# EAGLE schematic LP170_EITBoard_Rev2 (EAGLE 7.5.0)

## Sheet 1 of 9: Arduino Mega 2560 Board Connections
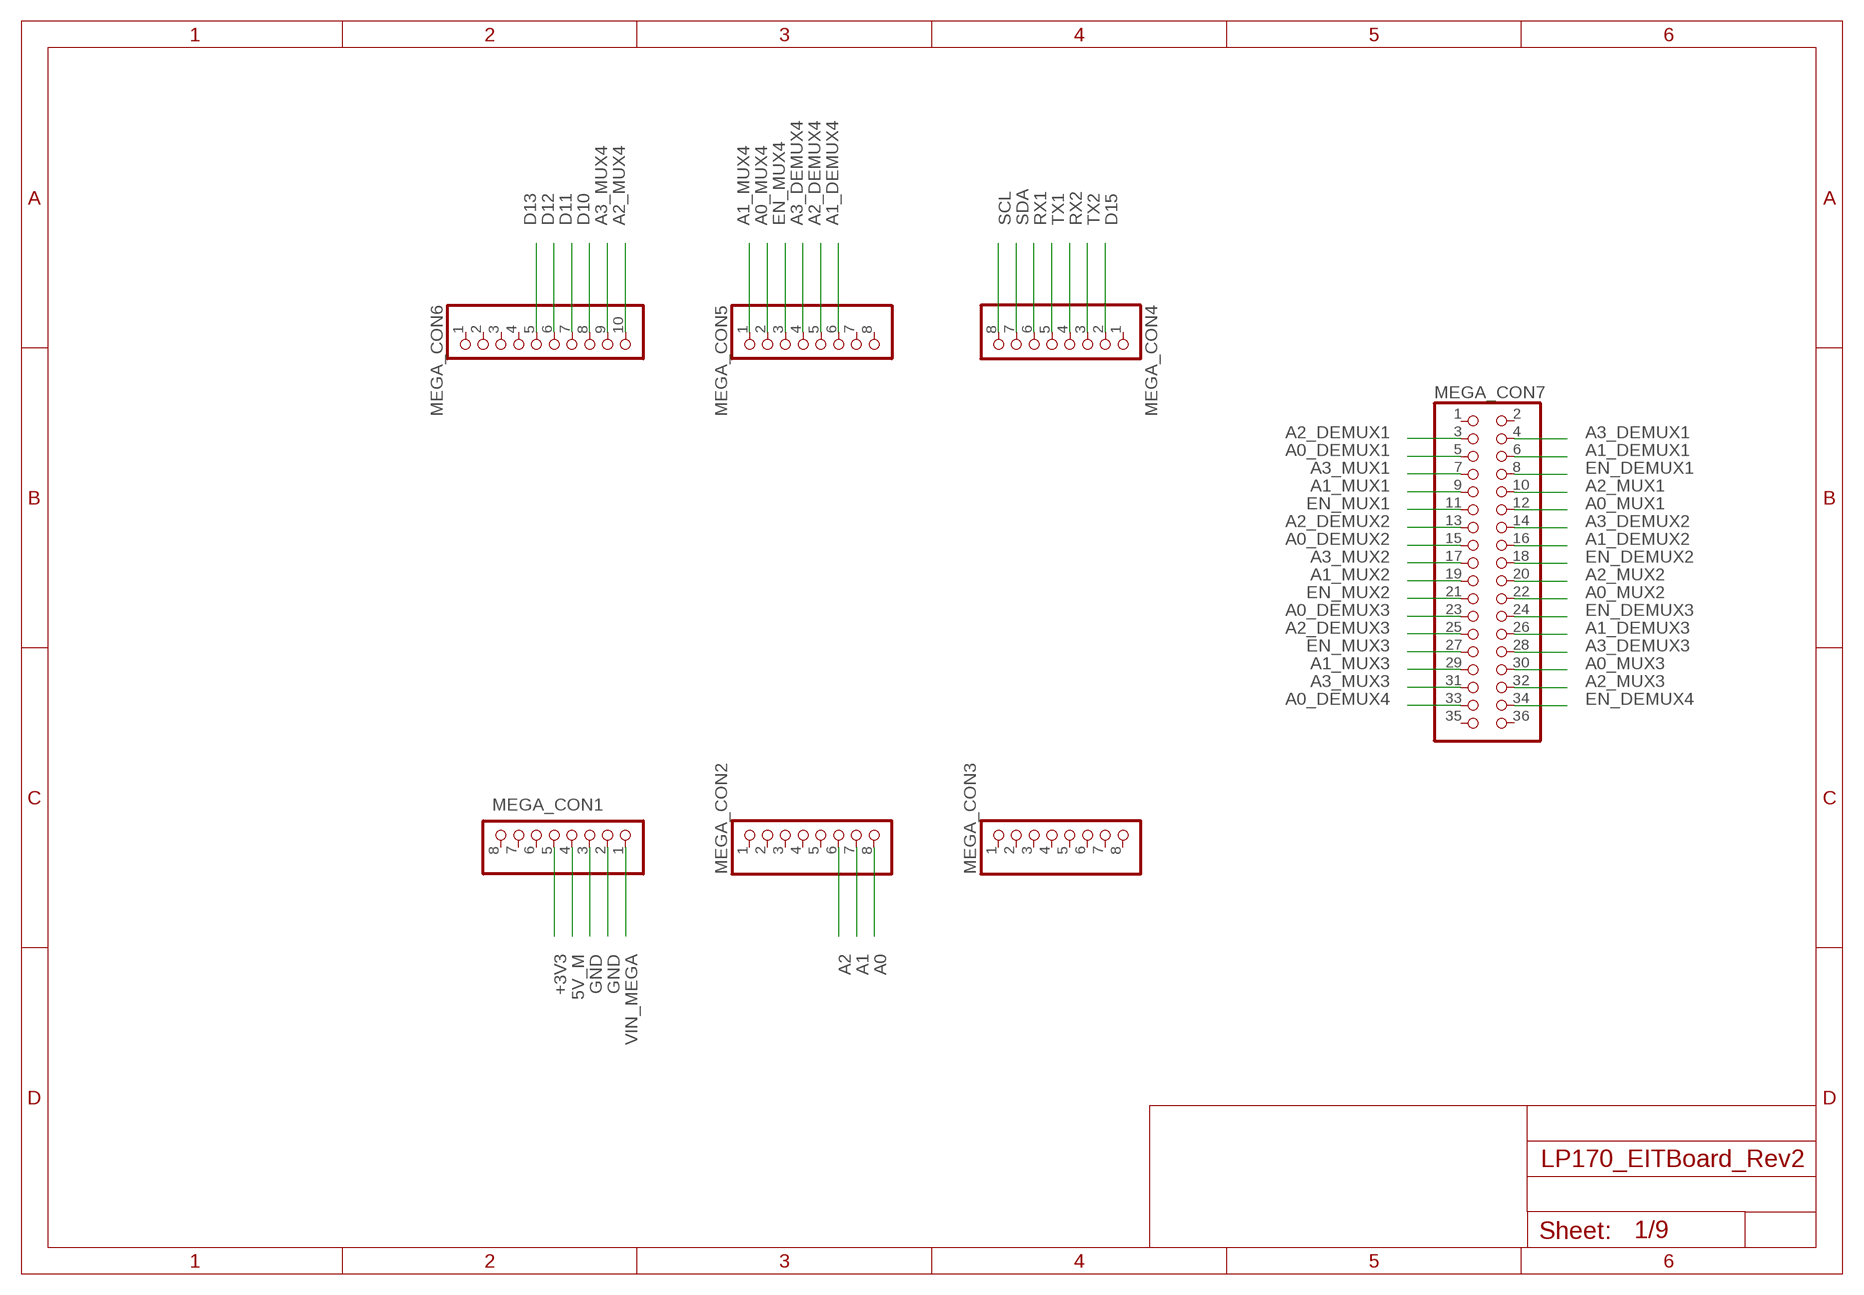
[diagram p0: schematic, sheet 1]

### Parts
MEGA_CON1  PINHD-1X8BIG  [1X08-BIG]
MEGA_CON2  PINHD-1X8BIG  [1X08-BIG]
MEGA_CON3  PINHD-1X8BIG  [1X08-BIG]
MEGA_CON4  PINHD-1X8BIG  [1X08-BIG]
MEGA_CON5  PINHD-1X8BIG  [1X08-BIG]
MEGA_CON6  PINHD-1X10  [1X10-BIG]
MEGA_CON7  PINHD-2X18  [2X18]

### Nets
5V_M: MEGA_CON1.4
+3V3: MEGA_CON1.5 ; also sheet 3,9
A0: MEGA_CON2.8
A0_DEMUX1: MEGA_CON7.5 ; also sheet 4
A0_DEMUX2: MEGA_CON7.15 ; also sheet 4
A0_DEMUX3: MEGA_CON7.23 ; also sheet 4
A0_DEMUX4: MEGA_CON7.33 ; also sheet 4
A0_MUX1: MEGA_CON7.12 ; also sheet 5
A0_MUX2: MEGA_CON7.22 ; also sheet 5
A0_MUX3: MEGA_CON7.30 ; also sheet 5
A0_MUX4: MEGA_CON5.2 ; also sheet 5
A1: MEGA_CON2.7
A1_DEMUX1: MEGA_CON7.6 ; also sheet 4
A1_DEMUX2: MEGA_CON7.16 ; also sheet 4
A1_DEMUX3: MEGA_CON7.26 ; also sheet 4
A1_DEMUX4: MEGA_CON5.6 ; also sheet 4
A1_MUX1: MEGA_CON7.9 ; also sheet 5
A1_MUX2: MEGA_CON7.19 ; also sheet 5
A1_MUX3: MEGA_CON7.29 ; also sheet 5
A1_MUX4: MEGA_CON5.1 ; also sheet 5
A2: MEGA_CON2.6
A2_DEMUX1: MEGA_CON7.3 ; also sheet 4
A2_DEMUX2: MEGA_CON7.13 ; also sheet 4
A2_DEMUX3: MEGA_CON7.25 ; also sheet 4
A2_DEMUX4: MEGA_CON5.5 ; also sheet 4
A2_MUX1: MEGA_CON7.10 ; also sheet 5
A2_MUX2: MEGA_CON7.20 ; also sheet 5
A2_MUX3: MEGA_CON7.32 ; also sheet 5
A2_MUX4: MEGA_CON6.10 ; also sheet 5
A3_DEMUX1: MEGA_CON7.4 ; also sheet 4
A3_DEMUX2: MEGA_CON7.14 ; also sheet 4
A3_DEMUX3: MEGA_CON7.28 ; also sheet 4
A3_DEMUX4: MEGA_CON5.4 ; also sheet 4
A3_MUX1: MEGA_CON7.7 ; also sheet 5
A3_MUX2: MEGA_CON7.17 ; also sheet 5
A3_MUX3: MEGA_CON7.31 ; also sheet 5
A3_MUX4: MEGA_CON6.9 ; also sheet 5
D10: MEGA_CON6.8
D11: MEGA_CON6.7
D12: MEGA_CON6.6
D13: MEGA_CON6.5
D15: MEGA_CON4.2 ; also sheet 9
EN_DEMUX1: MEGA_CON7.8 ; also sheet 4
EN_DEMUX2: MEGA_CON7.18 ; also sheet 4
EN_DEMUX3: MEGA_CON7.24 ; also sheet 4
EN_DEMUX4: MEGA_CON7.34 ; also sheet 4
EN_MUX1: MEGA_CON7.11 ; also sheet 5
EN_MUX2: MEGA_CON7.21 ; also sheet 5
EN_MUX3: MEGA_CON7.27 ; also sheet 5
EN_MUX4: MEGA_CON5.3 ; also sheet 5
GND: MEGA_CON1.2 MEGA_CON1.3 ; also sheet 2,3,4,5,6,7,9
RX1: MEGA_CON4.6
RX2: MEGA_CON4.4 ; also sheet 9
SCL: MEGA_CON4.8 ; also sheet 3
SDA: MEGA_CON4.7 ; also sheet 3
TX1: MEGA_CON4.5
TX2: MEGA_CON4.3 ; also sheet 9
VIN_MEGA: MEGA_CON1.1 ; also sheet 2
Unconnected: MEGA_CON1.6 MEGA_CON1.7 MEGA_CON1.8 MEGA_CON2.1 MEGA_CON2.2 MEGA_CON2.3 MEGA_CON2.4 MEGA_CON2.5 MEGA_CON3.1 MEGA_CON3.2 MEGA_CON3.3 MEGA_CON3.4 MEGA_CON3.5 MEGA_CON3.6 MEGA_CON3.7 MEGA_CON3.8 MEGA_CON4.1 MEGA_CON5.7 MEGA_CON5.8 MEGA_CON6.1 MEGA_CON6.2 MEGA_CON6.3 MEGA_CON6.4 MEGA_CON7.1 MEGA_CON7.2 MEGA_CON7.35 MEGA_CON7.36

## Sheet 2 of 9: Power Supply
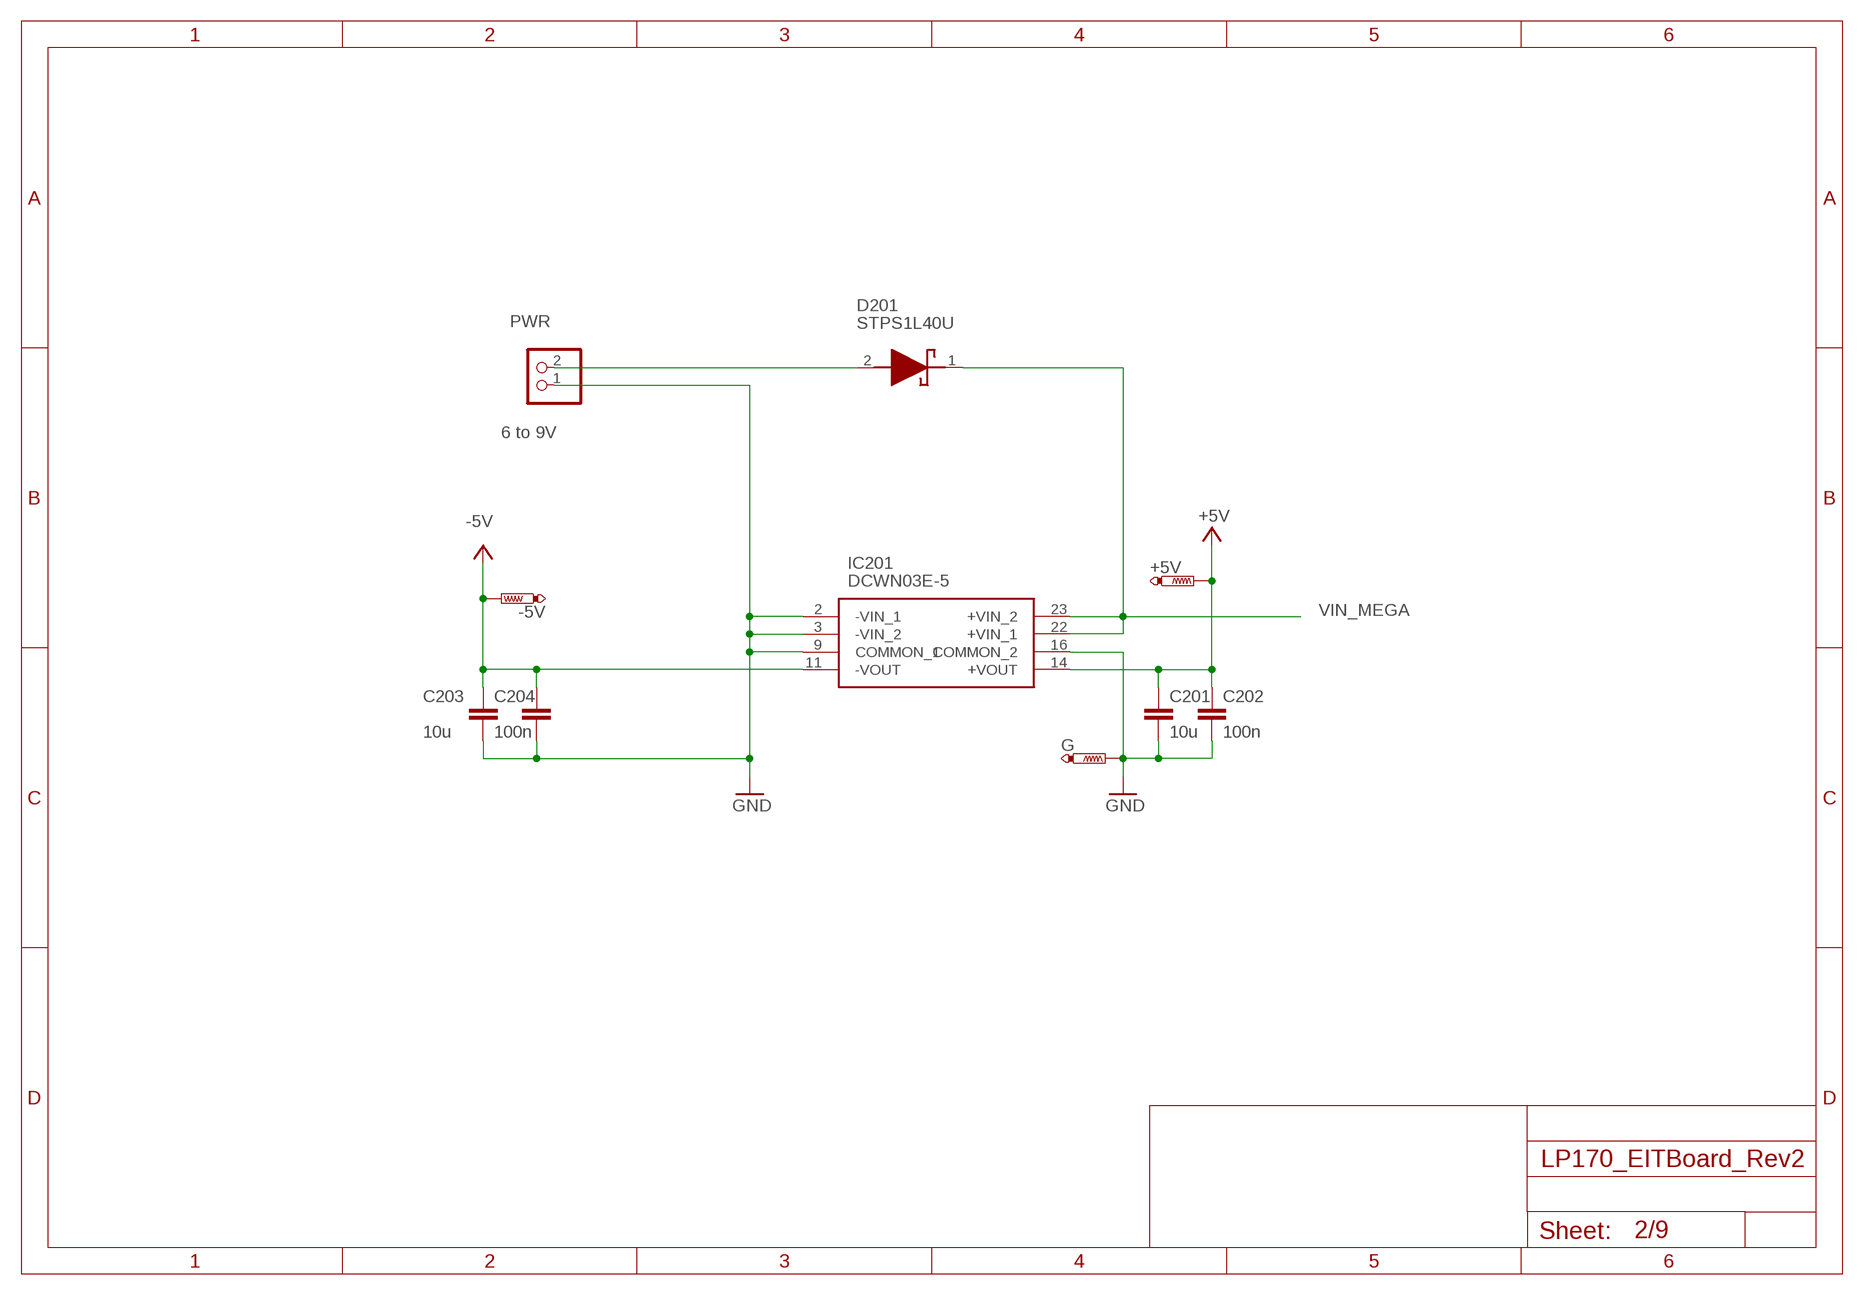
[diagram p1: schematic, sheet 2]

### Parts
+5V  PTR1B1,27  [B1,27]
-5V  PTR1B1,27  [B1,27]
C201  10u  C-EUC0805  [C0805]
C202  100n  C-EUC0805  [C0805]
C203  10u  C-EUC0805  [C0805]
C204  100n  C-EUC0805  [C0805]
D201  STPS1L40U  [DIOM5436X265N]
G  PTR1B1,27  [B1,27]
IC201  DCWN03E-5  DCWN03E-15  [DCWN03E15]
PWR  PINHD-1X02_2.54  [1X02]

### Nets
+5V: +5V.TP C201.1 C202.1 IC201.14(+VOUT) ; also sheet 3,4,5
-5V: -5V.TP C203.1 C204.1 IC201.11(-VOUT) ; also sheet 3,4,5
GND: C201.2 C202.2 C203.2 C204.2 G.TP IC201.2(-VIN_1) IC201.3(-VIN_2) IC201.9(COMMON_1) IC201.16(COMMON_2) PWR.1 ; also sheet 1,3,4,5,6,7,9
N$1: D201.2(A) PWR.2
VIN_MEGA: D201.1(K) IC201.22(+VIN_1) IC201.23(+VIN_2) ; also sheet 1

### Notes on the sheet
- 6 to 9V

## Sheet 3 of 9: Impedanz Converter
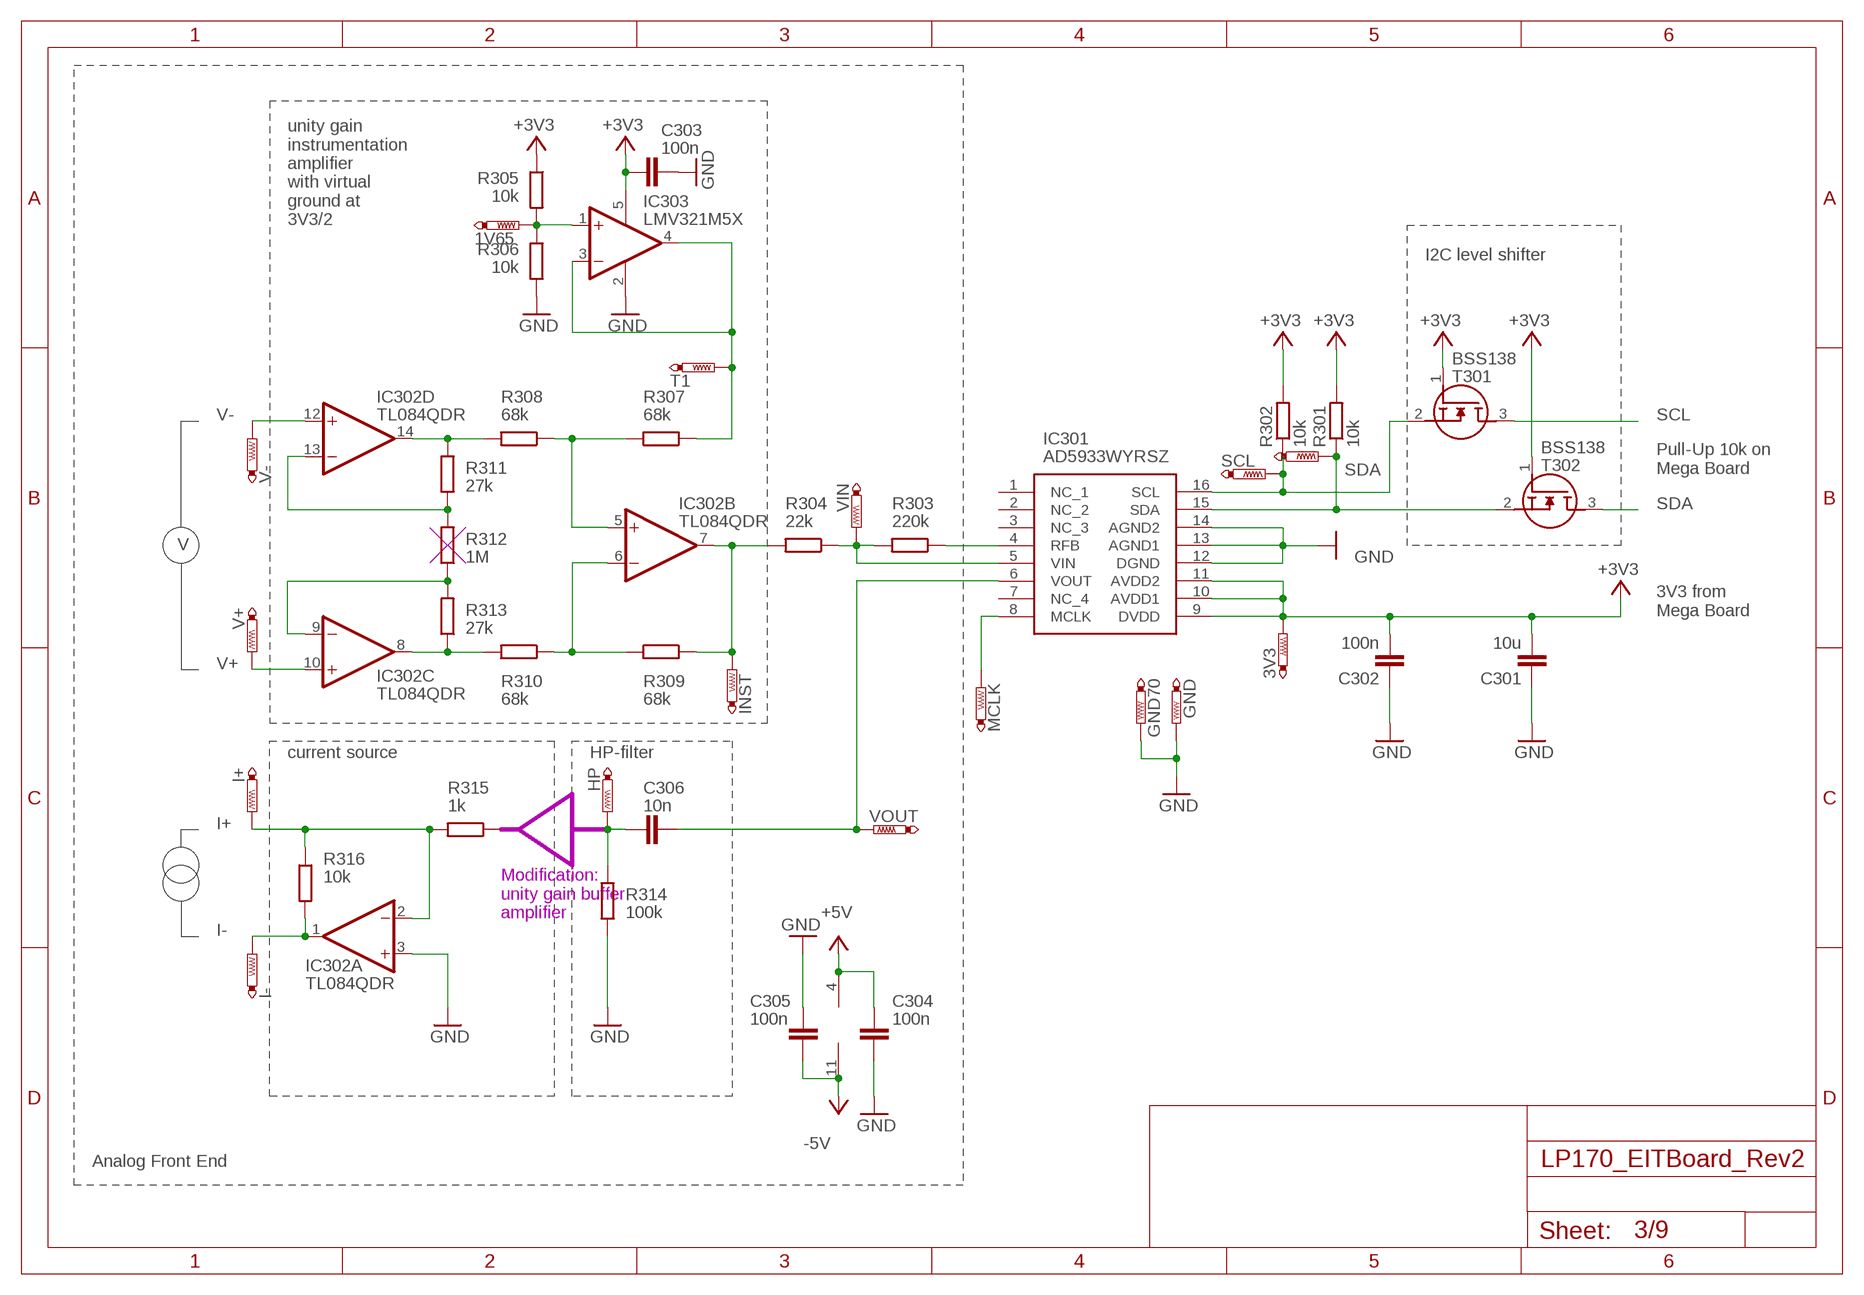
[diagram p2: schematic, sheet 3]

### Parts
1V65  PTR1B1,27  [B1,27]
3V3  PTR1B1,27  [B1,27]
C301  10u  C-EUC0805  [C0805]
C302  100n  C-EUC0805  [C0805]
C303  100n  C-EUC0805  [C0805]
C304  100n  C-EUC0805  [C0805]
C305  100n  C-EUC0805  [C0805]
C306  10n  C-EUC0805  [C0805]
GND  PTR1B1,27  [B1,27]
GND70  PTR1B1,27  [B1,27]
HP  PTR1B1,27  [B1,27]
I+  PTR1B1,27  [B1,27]
I-  PTR1B1,27  [B1,27]
IC301  AD5933WYRSZ  AD5933WYRSZ-REEL7  [SOP65P780X200-16N]
IC302  TL084QDR  TL084D  [SO14]
IC303  LMV321M5X  [SOT23-5]
INST  PTR1B1,27  [B1,27]
MCLK  PTR1B1,27  [B1,27]
R301  10k  R-EU_R0805  [R0805]
R302  10k  R-EU_R0805  [R0805]
R303  220k  R-EU_R0805  [R0805]
R304  22k  R-EU_R0805  [R0805]
R305  10k  R-EU_R0805  [R0805]
R306  10k  R-EU_R0805  [R0805]
R307  68k  R-EU_R0805  [R0805]
R308  68k  R-EU_R0805  [R0805]
R309  68k  R-EU_R0805  [R0805]
R310  68k  R-EU_R0805  [R0805]
R311  27k  R-EU_R0805  [R0805]
R312  1M  R-EU_R0805  [R0805]
R313  27k  R-EU_R0805  [R0805]
R314  100k  R-EU_R0805  [R0805]
R315  1k  R-EU_R0805  [R0805]
R316  10k  R-EU_R0805  [R0805]
SCL  PTR1B1,27  [B1,27]
SDA  PTR1B1,27  [B1,27]
T1  PTR1B1,27  [B1,27]
T301  BSS138  BSS138LT3G  [SOT96P237X111-3N]
T302  BSS138  BSS138LT3G  [SOT96P237X111-3N]
V+  PTR1B1,27  [B1,27]
V-  PTR1B1,27  [B1,27]
VIN  PTR1B1,27  [B1,27]
VOUT  PTR1B1,27  [B1,27]

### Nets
+3V3: 3V3.TP C301.2 C302.2 C303.2 IC301.9(DVDD) IC301.10(AVDD1) IC301.11(AVDD2) IC303.5(V+) R301.2 R302.2 R305.1 T301.1(G) T302.1(G) ; also sheet 1,9
+5V: C304.2 IC302.4(P:V+) ; also sheet 2,4,5
-5V: C305.2 IC302.11(P:V-) ; also sheet 2,4,5
GND: C301.1 C302.1 C303.1 C304.1 C305.1 GND70.TP GND.TP IC301.12(DGND) IC301.13(AGND1) IC301.14(AGND2) IC302.3(A:+IN) IC303.2(V-) R306.2 R314.2 ; also sheet 1,2,4,5,6,7,9
I+: I+.TP IC302.2(A:-IN) R315.2 R316.1 ; also sheet 4
I-: I-.TP IC302.1(A:OUT) R316.2 ; also sheet 4
N$3: IC301.16(SCL) R302.1 SCL.TP T301.2(S)
N$5: IC301.15(SDA) R301.1 SDA.TP T302.2(S)
N$7: IC301.4(RFB) R303.1
N$8: IC301.5(VIN) R303.2 R304.1 VIN.TP
N$9: IC302.7(B:OUT) INST.TP R304.2 R309.1
N$10: 1V65.TP IC303.1(+IN) R305.2 R306.1
N$11: IC302.5(B:+IN) R307.2 R308.1
N$12: C306.1 IC301.6(VOUT) VOUT.TP
N$13: IC303.3(-IN) IC303.4(OUT) R307.1 T1.TP
N$14: IC302.6(B:-IN) R309.2 R310.1
N$15: IC302.8(C:OUT) R310.2 R313.1
N$16: IC302.14(D:OUT) R308.2 R311.2
N$17: IC302.13(D:-IN) R311.1 R312.2
N$18: IC302.9(C:-IN) R312.1 R313.2
N$19: C306.2 HP.TP R314.1
N$90: IC301.8(MCLK) MCLK.TP
SCL: T301.3(D) ; also sheet 1
SDA: T302.3(D) ; also sheet 1
V+: IC302.10(C:+IN) V+.TP ; also sheet 5
V-: IC302.12(D:+IN) V-.TP ; also sheet 5
Unconnected: IC301.1(NC_1) IC301.2(NC_2) IC301.3(NC_3) IC301.7(NC_4) R315.1

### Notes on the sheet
- unity gain  
  instrumentation
  amplifier
  with virtual
  ground at
  3V3/2
- I2C level shifter
- Pull-Up 10k on
  Mega Board
- V
- 3V3 from
  Mega Board
- current source | HP-filter
- Modification: 
  unity gain buffer 
  amplifier
- Analog Front End

## Sheet 4 of 9: Demultiplexer - Current Source
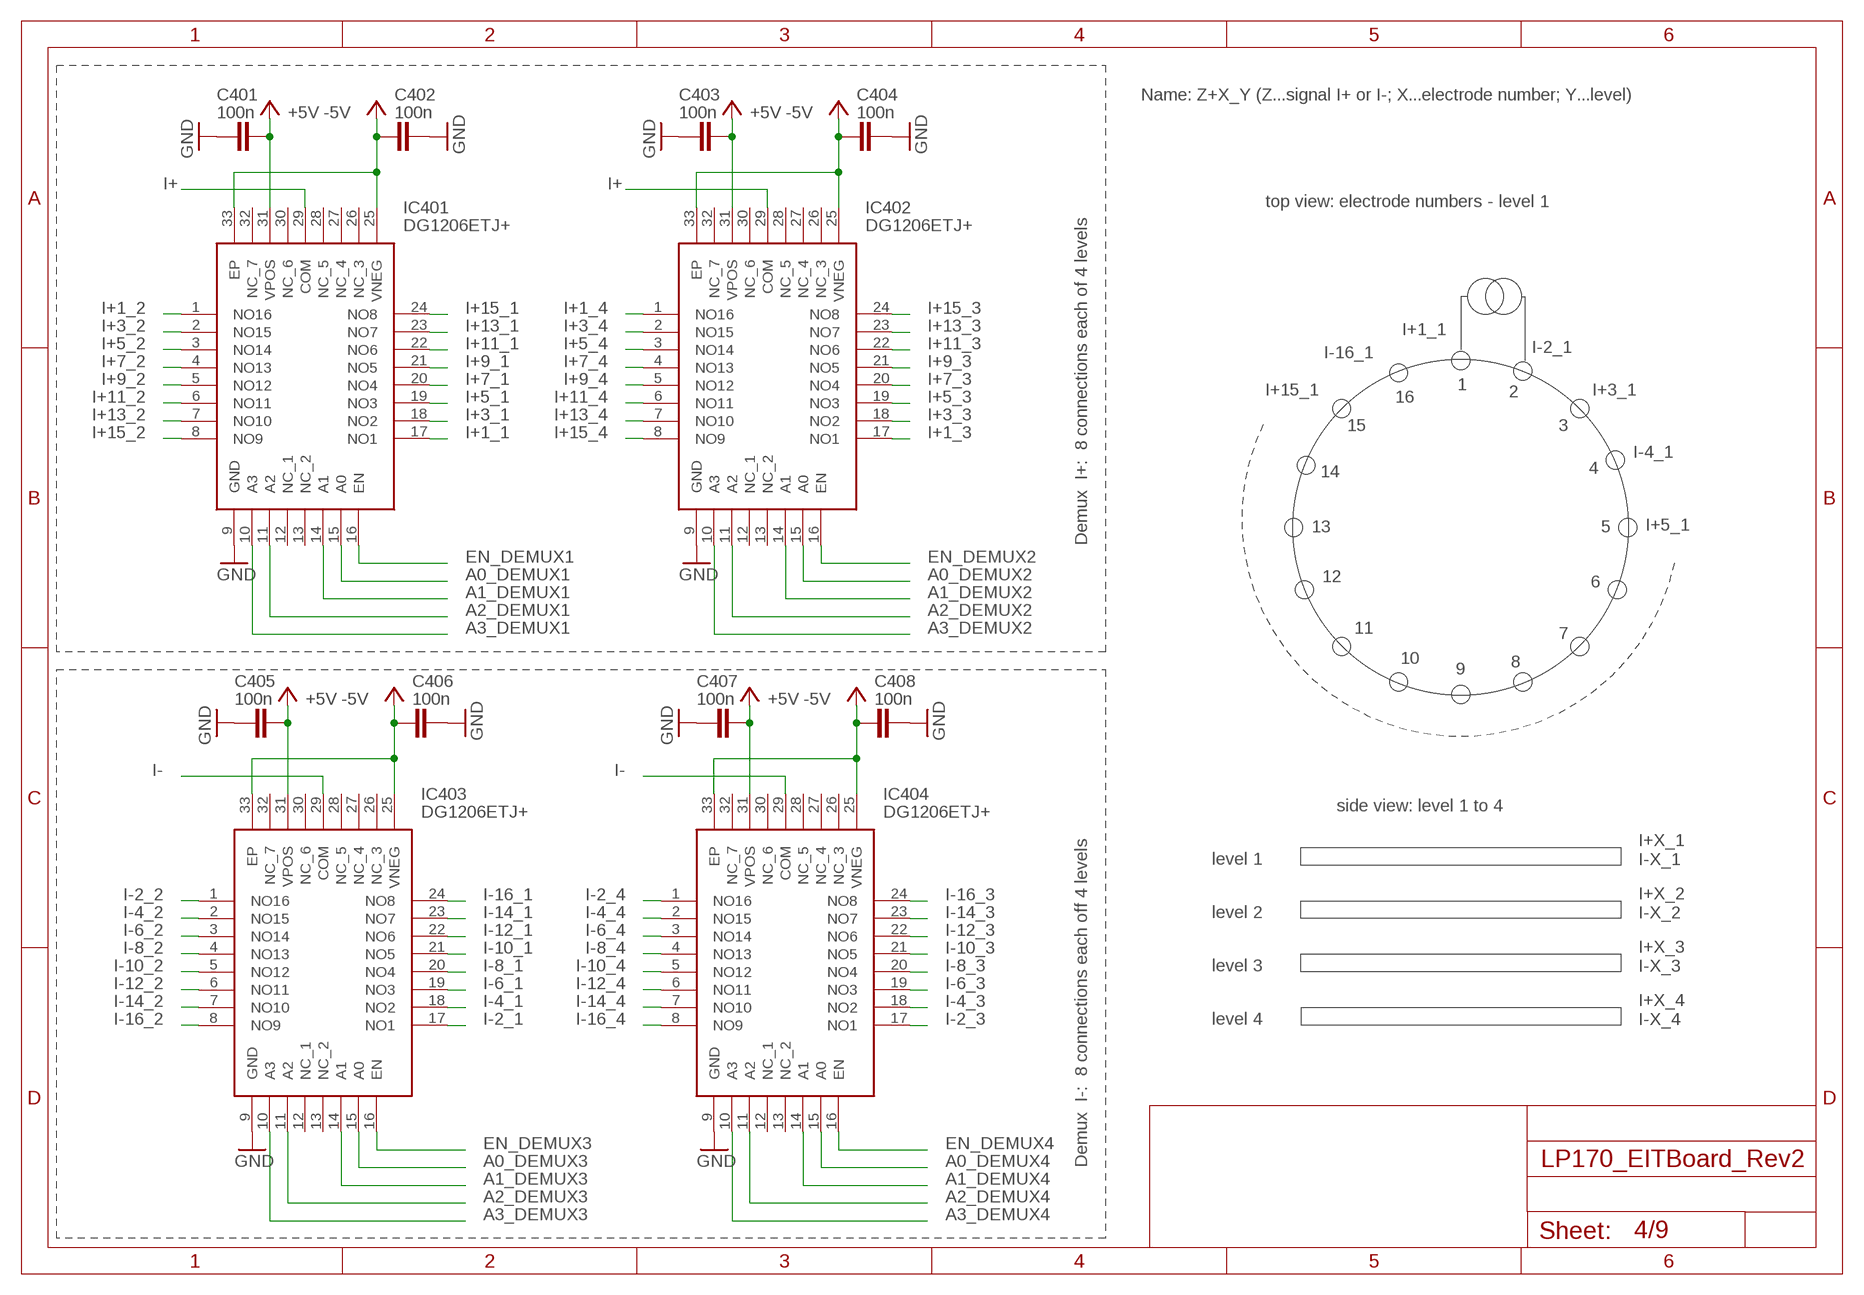
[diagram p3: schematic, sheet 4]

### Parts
C401  100n  C-EUC0805  [C0805]
C402  100n  C-EUC0805  [C0805]
C403  100n  C-EUC0805  [C0805]
C404  100n  C-EUC0805  [C0805]
C405  100n  C-EUC0805  [C0805]
C406  100n  C-EUC0805  [C0805]
C407  100n  C-EUC0805  [C0805]
C408  100n  C-EUC0805  [C0805]
IC401  DG1206ETJ+  [QFN50P500X500X80-33N]
IC402  DG1206ETJ+  [QFN50P500X500X80-33N]
IC403  DG1206ETJ+  [QFN50P500X500X80-33N]
IC404  DG1206ETJ+  [QFN50P500X500X80-33N]

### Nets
+5V: C401.2 C403.2 C405.2 C407.2 IC401.31(VPOS) IC402.31(VPOS) IC403.31(VPOS) IC404.31(VPOS) ; also sheet 2,3,5
-5V: C402.2 C404.2 C406.2 C408.2 IC401.25(VNEG) IC401.33(EP) IC402.25(VNEG) IC402.33(EP) IC403.25(VNEG) IC403.33(EP) IC404.25(VNEG) IC404.33(EP) ; also sheet 2,3,5
A0_DEMUX1: IC401.15(A0) ; also sheet 1
A0_DEMUX2: IC402.15(A0) ; also sheet 1
A0_DEMUX3: IC403.15(A0) ; also sheet 1
A0_DEMUX4: IC404.15(A0) ; also sheet 1
A1_DEMUX1: IC401.14(A1) ; also sheet 1
A1_DEMUX2: IC402.14(A1) ; also sheet 1
A1_DEMUX3: IC403.14(A1) ; also sheet 1
A1_DEMUX4: IC404.14(A1) ; also sheet 1
A2_DEMUX1: IC401.11(A2) ; also sheet 1
A2_DEMUX2: IC402.11(A2) ; also sheet 1
A2_DEMUX3: IC403.11(A2) ; also sheet 1
A2_DEMUX4: IC404.11(A2) ; also sheet 1
A3_DEMUX1: IC401.10(A3) ; also sheet 1
A3_DEMUX2: IC402.10(A3) ; also sheet 1
A3_DEMUX3: IC403.10(A3) ; also sheet 1
A3_DEMUX4: IC404.10(A3) ; also sheet 1
EN_DEMUX1: IC401.16(EN) ; also sheet 1
EN_DEMUX2: IC402.16(EN) ; also sheet 1
EN_DEMUX3: IC403.16(EN) ; also sheet 1
EN_DEMUX4: IC404.16(EN) ; also sheet 1
GND: C401.1 C402.1 C403.1 C404.1 C405.1 C406.1 C407.1 C408.1 IC401.9(GND) IC402.9(GND) IC403.9(GND) IC404.9(GND) ; also sheet 1,2,3,5,6,7,9
I+: IC401.29(COM) IC402.29(COM) ; also sheet 3
I+1_1: IC401.17(NO1) ; also sheet 6
I+1_2: IC401.1(NO16) ; also sheet 6
I+1_3: IC402.17(NO1) ; also sheet 6
I+1_4: IC402.1(NO16) ; also sheet 6
I+3_1: IC401.18(NO2) ; also sheet 6
I+3_2: IC401.2(NO15) ; also sheet 6
I+3_3: IC402.18(NO2) ; also sheet 6
I+3_4: IC402.2(NO15) ; also sheet 6
I+5_1: IC401.19(NO3) ; also sheet 6
I+5_2: IC401.3(NO14) ; also sheet 6
I+5_3: IC402.19(NO3) ; also sheet 6
I+5_4: IC402.3(NO14) ; also sheet 6
I+7_1: IC401.20(NO4) ; also sheet 6
I+7_2: IC401.4(NO13) ; also sheet 6
I+7_3: IC402.20(NO4) ; also sheet 6
I+7_4: IC402.4(NO13) ; also sheet 6
I+9_1: IC401.21(NO5) ; also sheet 6
I+9_2: IC401.5(NO12) ; also sheet 6
I+9_3: IC402.21(NO5) ; also sheet 6
I+9_4: IC402.5(NO12) ; also sheet 6
I+11_1: IC401.22(NO6) ; also sheet 6
I+11_2: IC401.6(NO11) ; also sheet 6
I+11_3: IC402.22(NO6) ; also sheet 6
I+11_4: IC402.6(NO11) ; also sheet 6
I+13_1: IC401.23(NO7) ; also sheet 6
I+13_2: IC401.7(NO10) ; also sheet 6
I+13_3: IC402.23(NO7) ; also sheet 6
I+13_4: IC402.7(NO10) ; also sheet 6
I+15_1: IC401.24(NO8) ; also sheet 6
I+15_2: IC401.8(NO9) ; also sheet 6
I+15_3: IC402.24(NO8) ; also sheet 6
I+15_4: IC402.8(NO9) ; also sheet 6
I-: IC403.29(COM) IC404.29(COM) ; also sheet 3
I-2_1: IC403.17(NO1) ; also sheet 7
I-2_2: IC403.1(NO16) ; also sheet 7
I-2_3: IC404.17(NO1) ; also sheet 7
I-2_4: IC404.1(NO16) ; also sheet 7
I-4_1: IC403.18(NO2) ; also sheet 7
I-4_2: IC403.2(NO15) ; also sheet 7
I-4_3: IC404.18(NO2) ; also sheet 7
I-4_4: IC404.2(NO15) ; also sheet 7
I-6_1: IC403.19(NO3) ; also sheet 7
I-6_2: IC403.3(NO14) ; also sheet 7
I-6_3: IC404.19(NO3) ; also sheet 7
I-6_4: IC404.3(NO14) ; also sheet 7
I-8_1: IC403.20(NO4) ; also sheet 7
I-8_2: IC403.4(NO13) ; also sheet 7
I-8_3: IC404.20(NO4) ; also sheet 7
I-8_4: IC404.4(NO13) ; also sheet 7
I-10_1: IC403.21(NO5) ; also sheet 7
I-10_2: IC403.5(NO12) ; also sheet 7
I-10_3: IC404.21(NO5) ; also sheet 7
I-10_4: IC404.5(NO12) ; also sheet 7
I-12_1: IC403.22(NO6) ; also sheet 7
I-12_2: IC403.6(NO11) ; also sheet 7
I-12_3: IC404.22(NO6) ; also sheet 7
I-12_4: IC404.6(NO11) ; also sheet 7
I-14_1: IC403.23(NO7) ; also sheet 7
I-14_2: IC403.7(NO10) ; also sheet 7
I-14_3: IC404.23(NO7) ; also sheet 7
I-14_4: IC404.7(NO10) ; also sheet 7
I-16_1: IC403.24(NO8) ; also sheet 7
I-16_2: IC403.8(NO9) ; also sheet 7
I-16_3: IC404.24(NO8) ; also sheet 7
I-16_4: IC404.8(NO9) ; also sheet 7
Unconnected: IC401.12(NC_1) IC401.13(NC_2) IC401.26(NC_3) IC401.27(NC_4) IC401.28(NC_5) IC401.30(NC_6) IC401.32(NC_7) IC402.12(NC_1) IC402.13(NC_2) IC402.26(NC_3) IC402.27(NC_4) IC402.28(NC_5) IC402.30(NC_6) IC402.32(NC_7) IC403.12(NC_1) IC403.13(NC_2) IC403.26(NC_3) IC403.27(NC_4) IC403.28(NC_5) IC403.30(NC_6) IC403.32(NC_7) IC404.12(NC_1) IC404.13(NC_2) IC404.26(NC_3) IC404.27(NC_4) IC404.28(NC_5) IC404.30(NC_6) IC404.32(NC_7)

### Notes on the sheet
- Name: Z+X_Y (Z...signal I+ or I-; X...electrode number; Y...level)
- top view: electrode numbers - level 1
- I+1_1
- I-2_1
- I-16_1
- 1
- I+15_1 | 2 | I+3_1
- 16
- 15 | 3
- I-4_1
- 14 | 4
- 13 | 5 | I+5_1
- Demux  I+:  8 connections each of 4 levels
- 12
- 6
- 11
- 7
- 10 | 8
- 9
- side view: level 1 to 4
- level 1
- I+X_1
  I-X_1
- level 2
- I+X_2
  I-X_2
- level 3
- I+X_3
  I-X_3
- level 4
- I+X_4
  I-X_4
- Demux  I-:  8 connections each off 4 levels

## Sheet 5 of 9: Multiplexer - Voltage measurement
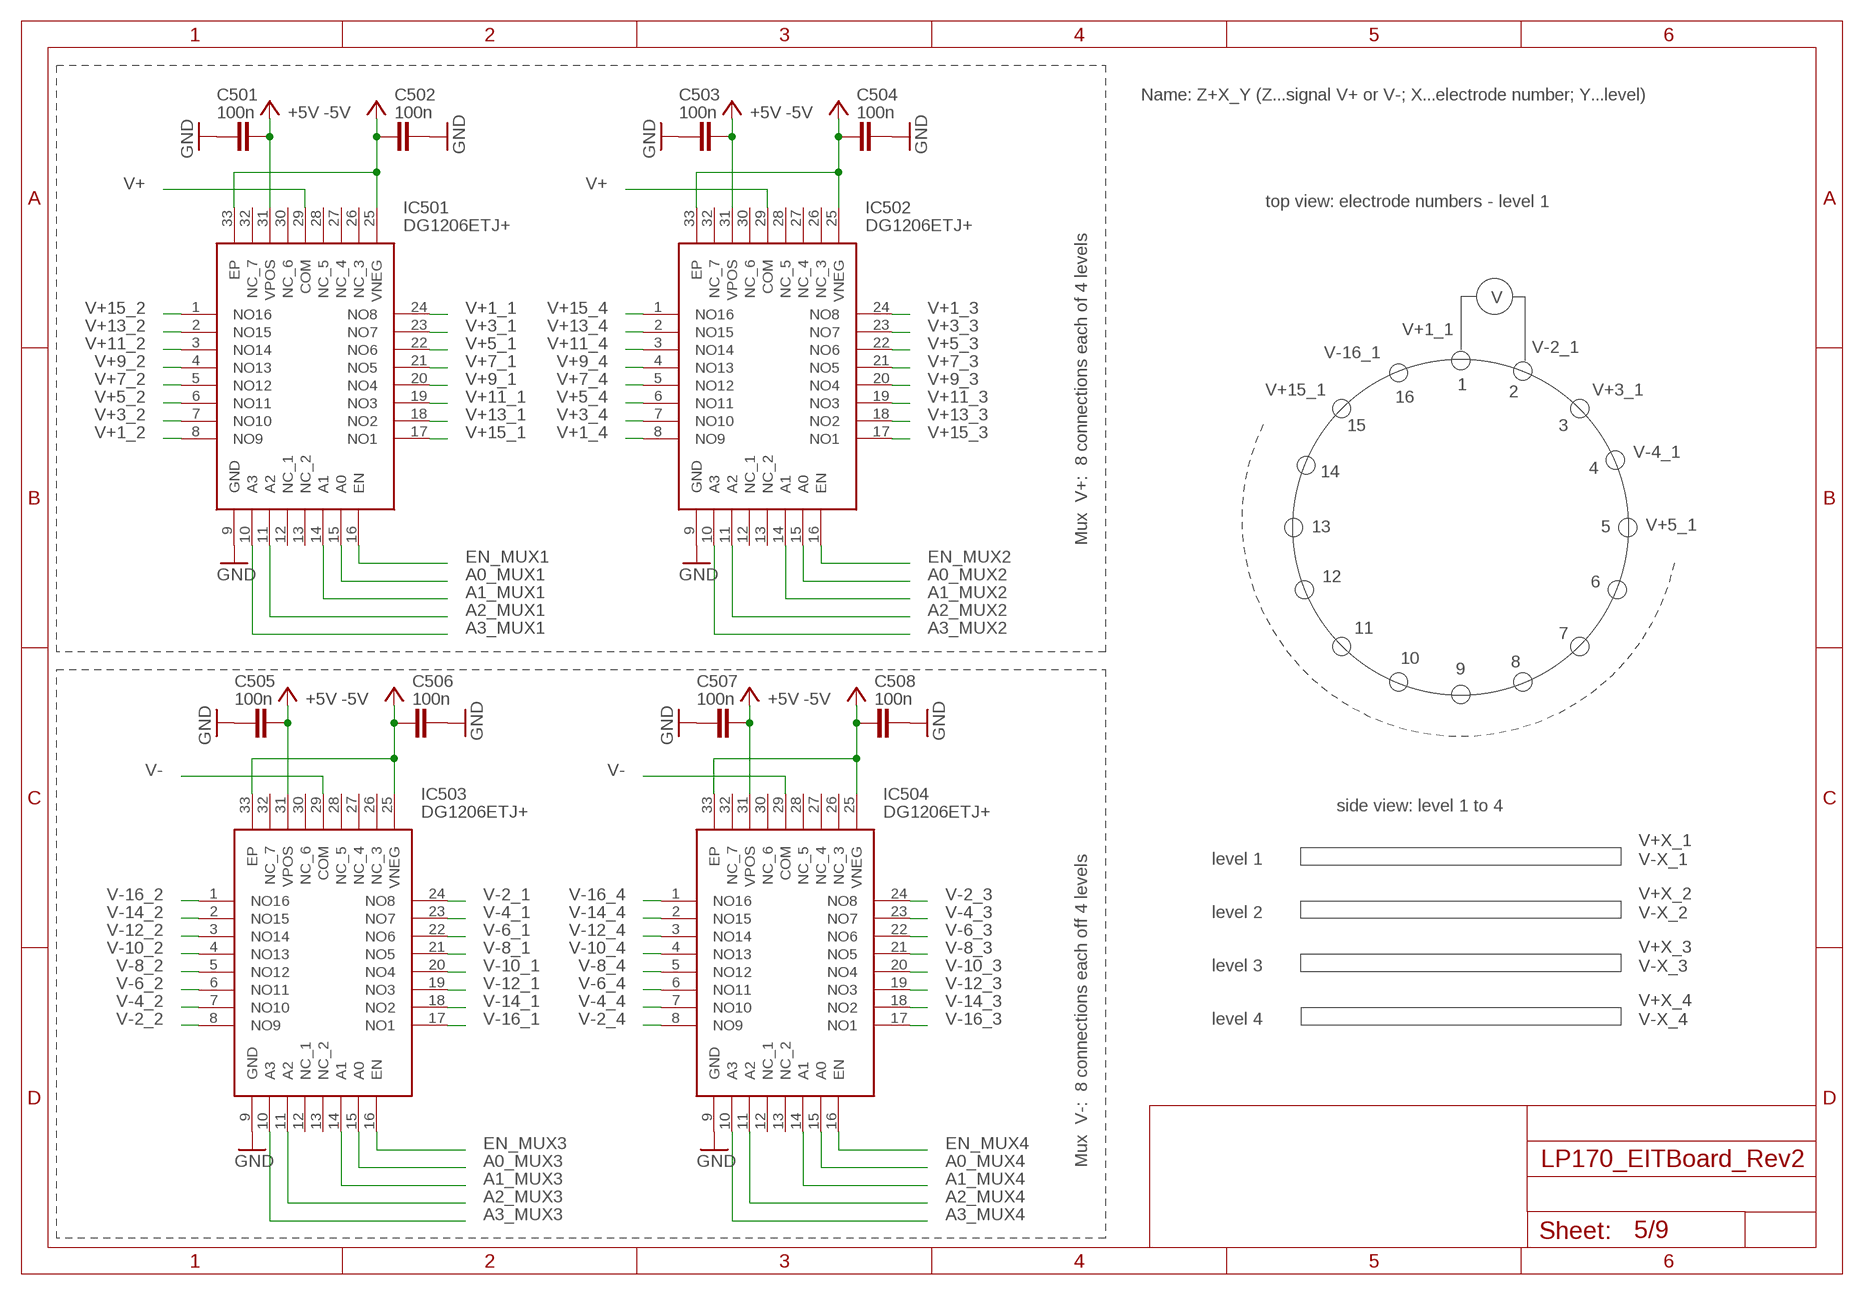
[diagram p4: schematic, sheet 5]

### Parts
C501  100n  C-EUC0805  [C0805]
C502  100n  C-EUC0805  [C0805]
C503  100n  C-EUC0805  [C0805]
C504  100n  C-EUC0805  [C0805]
C505  100n  C-EUC0805  [C0805]
C506  100n  C-EUC0805  [C0805]
C507  100n  C-EUC0805  [C0805]
C508  100n  C-EUC0805  [C0805]
IC501  DG1206ETJ+  [QFN50P500X500X80-33N]
IC502  DG1206ETJ+  [QFN50P500X500X80-33N]
IC503  DG1206ETJ+  [QFN50P500X500X80-33N]
IC504  DG1206ETJ+  [QFN50P500X500X80-33N]

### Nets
+5V: C501.2 C503.2 C505.2 C507.2 IC501.31(VPOS) IC502.31(VPOS) IC503.31(VPOS) IC504.31(VPOS) ; also sheet 2,3,4
-5V: C502.2 C504.2 C506.2 C508.2 IC501.25(VNEG) IC501.33(EP) IC502.25(VNEG) IC502.33(EP) IC503.25(VNEG) IC503.33(EP) IC504.25(VNEG) IC504.33(EP) ; also sheet 2,3,4
A0_MUX1: IC501.15(A0) ; also sheet 1
A0_MUX2: IC502.15(A0) ; also sheet 1
A0_MUX3: IC503.15(A0) ; also sheet 1
A0_MUX4: IC504.15(A0) ; also sheet 1
A1_MUX1: IC501.14(A1) ; also sheet 1
A1_MUX2: IC502.14(A1) ; also sheet 1
A1_MUX3: IC503.14(A1) ; also sheet 1
A1_MUX4: IC504.14(A1) ; also sheet 1
A2_MUX1: IC501.11(A2) ; also sheet 1
A2_MUX2: IC502.11(A2) ; also sheet 1
A2_MUX3: IC503.11(A2) ; also sheet 1
A2_MUX4: IC504.11(A2) ; also sheet 1
A3_MUX1: IC501.10(A3) ; also sheet 1
A3_MUX2: IC502.10(A3) ; also sheet 1
A3_MUX3: IC503.10(A3) ; also sheet 1
A3_MUX4: IC504.10(A3) ; also sheet 1
EN_MUX1: IC501.16(EN) ; also sheet 1
EN_MUX2: IC502.16(EN) ; also sheet 1
EN_MUX3: IC503.16(EN) ; also sheet 1
EN_MUX4: IC504.16(EN) ; also sheet 1
GND: C501.1 C502.1 C503.1 C504.1 C505.1 C506.1 C507.1 C508.1 IC501.9(GND) IC502.9(GND) IC503.9(GND) IC504.9(GND) ; also sheet 1,2,3,4,6,7,9
V+: IC501.29(COM) IC502.29(COM) ; also sheet 3
V+1_1: IC501.24(NO8) ; also sheet 6
V+1_2: IC501.8(NO9) ; also sheet 6
V+1_3: IC502.24(NO8) ; also sheet 6
V+1_4: IC502.8(NO9) ; also sheet 6
V+3_1: IC501.23(NO7) ; also sheet 6
V+3_2: IC501.7(NO10) ; also sheet 6
V+3_3: IC502.23(NO7) ; also sheet 6
V+3_4: IC502.7(NO10) ; also sheet 6
V+5_1: IC501.22(NO6) ; also sheet 6
V+5_2: IC501.6(NO11) ; also sheet 6
V+5_3: IC502.22(NO6) ; also sheet 6
V+5_4: IC502.6(NO11) ; also sheet 6
V+7_1: IC501.21(NO5) ; also sheet 6
V+7_2: IC501.5(NO12) ; also sheet 6
V+7_3: IC502.21(NO5) ; also sheet 6
V+7_4: IC502.5(NO12) ; also sheet 6
V+9_1: IC501.20(NO4) ; also sheet 6
V+9_2: IC501.4(NO13) ; also sheet 6
V+9_3: IC502.20(NO4) ; also sheet 6
V+9_4: IC502.4(NO13) ; also sheet 6
V+11_1: IC501.19(NO3) ; also sheet 6
V+11_2: IC501.3(NO14) ; also sheet 6
V+11_3: IC502.19(NO3) ; also sheet 6
V+11_4: IC502.3(NO14) ; also sheet 6
V+13_1: IC501.18(NO2) ; also sheet 6
V+13_2: IC501.2(NO15) ; also sheet 6
V+13_3: IC502.18(NO2) ; also sheet 6
V+13_4: IC502.2(NO15) ; also sheet 6
V+15_1: IC501.17(NO1) ; also sheet 6
V+15_2: IC501.1(NO16) ; also sheet 6
V+15_3: IC502.17(NO1) ; also sheet 6
V+15_4: IC502.1(NO16) ; also sheet 6
V-: IC503.29(COM) IC504.29(COM) ; also sheet 3
V-2_1: IC503.24(NO8) ; also sheet 7
V-2_2: IC503.8(NO9) ; also sheet 7
V-2_3: IC504.24(NO8) ; also sheet 7
V-2_4: IC504.8(NO9) ; also sheet 7
V-4_1: IC503.23(NO7) ; also sheet 7
V-4_2: IC503.7(NO10) ; also sheet 7
V-4_3: IC504.23(NO7) ; also sheet 7
V-4_4: IC504.7(NO10) ; also sheet 7
V-6_1: IC503.22(NO6) ; also sheet 7
V-6_2: IC503.6(NO11) ; also sheet 7
V-6_3: IC504.22(NO6) ; also sheet 7
V-6_4: IC504.6(NO11) ; also sheet 7
V-8_1: IC503.21(NO5) ; also sheet 7
V-8_2: IC503.5(NO12) ; also sheet 7
V-8_3: IC504.21(NO5) ; also sheet 7
V-8_4: IC504.5(NO12) ; also sheet 7
V-10_1: IC503.20(NO4) ; also sheet 7
V-10_2: IC503.4(NO13) ; also sheet 7
V-10_3: IC504.20(NO4) ; also sheet 7
V-10_4: IC504.4(NO13) ; also sheet 7
V-12_1: IC503.19(NO3) ; also sheet 7
V-12_2: IC503.3(NO14) ; also sheet 7
V-12_3: IC504.19(NO3) ; also sheet 7
V-12_4: IC504.3(NO14) ; also sheet 7
V-14_1: IC503.18(NO2) ; also sheet 7
V-14_2: IC503.2(NO15) ; also sheet 7
V-14_3: IC504.18(NO2) ; also sheet 7
V-14_4: IC504.2(NO15) ; also sheet 7
V-16_1: IC503.17(NO1) ; also sheet 7
V-16_2: IC503.1(NO16) ; also sheet 7
V-16_3: IC504.17(NO1) ; also sheet 7
V-16_4: IC504.1(NO16) ; also sheet 7
Unconnected: IC501.12(NC_1) IC501.13(NC_2) IC501.26(NC_3) IC501.27(NC_4) IC501.28(NC_5) IC501.30(NC_6) IC501.32(NC_7) IC502.12(NC_1) IC502.13(NC_2) IC502.26(NC_3) IC502.27(NC_4) IC502.28(NC_5) IC502.30(NC_6) IC502.32(NC_7) IC503.12(NC_1) IC503.13(NC_2) IC503.26(NC_3) IC503.27(NC_4) IC503.28(NC_5) IC503.30(NC_6) IC503.32(NC_7) IC504.12(NC_1) IC504.13(NC_2) IC504.26(NC_3) IC504.27(NC_4) IC504.28(NC_5) IC504.30(NC_6) IC504.32(NC_7)

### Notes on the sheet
- Name: Z+X_Y (Z...signal V+ or V-; X...electrode number; Y...level)
- top view: electrode numbers - level 1
- V
- V+1_1
- V-2_1
- V-16_1
- 1
- V+15_1 | 2 | V+3_1
- 16
- 15 | 3
- V-4_1
- 14 | 4
- 13 | 5 | V+5_1
- Mux  V+:  8 connections each of 4 levels
- 12
- 6
- 11
- 7
- 10 | 8
- 9
- side view: level 1 to 4
- level 1
- V+X_1
  V-X_1
- level 2
- V+X_2
  V-X_2
- level 3
- V+X_3
  V-X_3
- level 4
- V+X_4
  V-X_4
- Mux  V-:  8 connections each off 4 levels

## Sheet 6 of 9: Electrode Connections I+ and V+
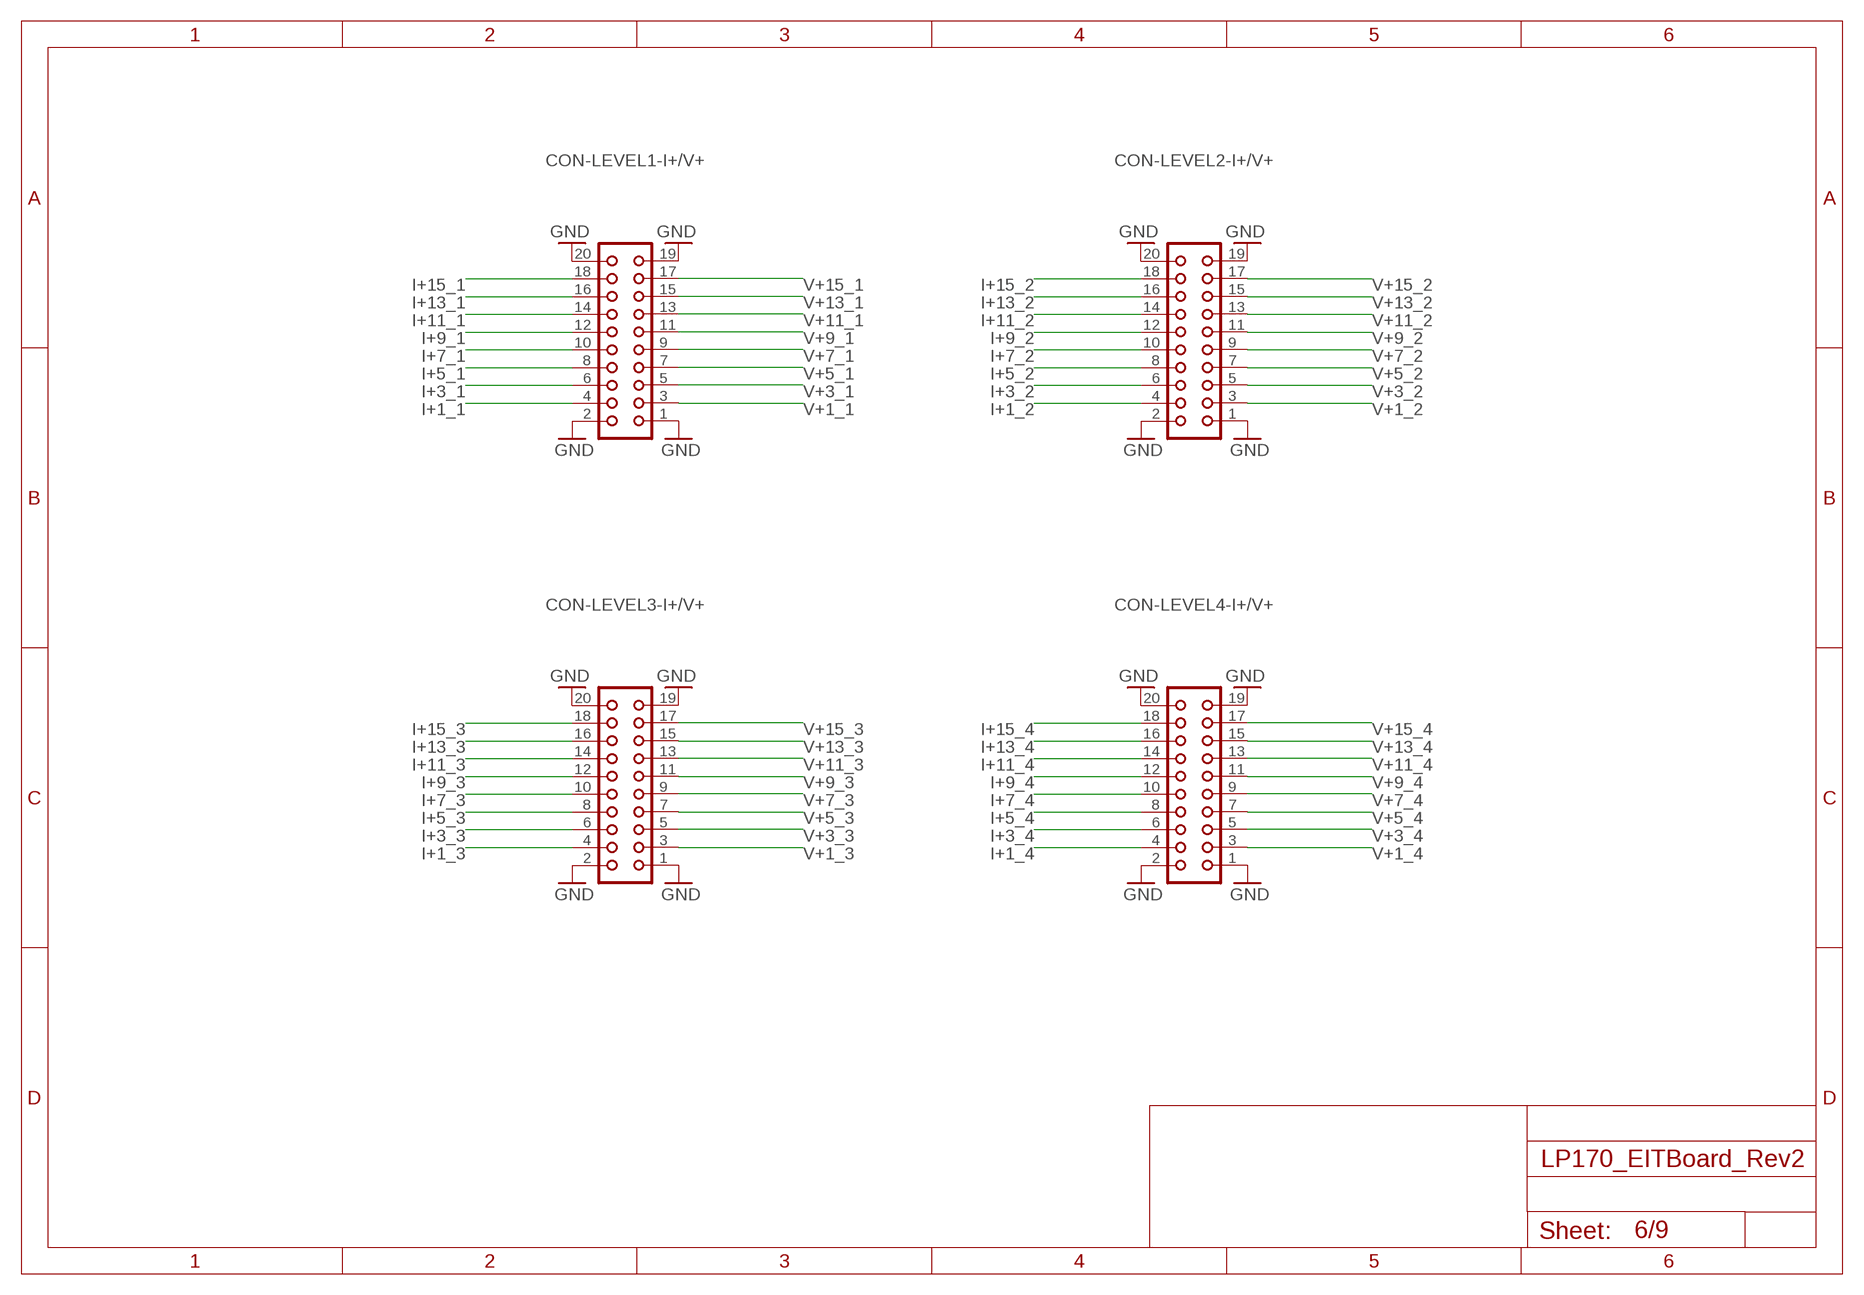
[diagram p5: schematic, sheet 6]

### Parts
CON-LEVEL1-I+/V+  CON20  [CON20]
CON-LEVEL2-I+/V+  CON20  [CON20]
CON-LEVEL3-I+/V+  CON20  [CON20]
CON-LEVEL4-I+/V+  CON20  [CON20]

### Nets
GND: CON-LEVEL1-I+/V+.1 CON-LEVEL1-I+/V+.2 CON-LEVEL1-I+/V+.19 CON-LEVEL1-I+/V+.20 CON-LEVEL2-I+/V+.1 CON-LEVEL2-I+/V+.2 CON-LEVEL2-I+/V+.19 CON-LEVEL2-I+/V+.20 CON-LEVEL3-I+/V+.1 CON-LEVEL3-I+/V+.2 CON-LEVEL3-I+/V+.19 CON-LEVEL3-I+/V+.20 CON-LEVEL4-I+/V+.1 CON-LEVEL4-I+/V+.2 CON-LEVEL4-I+/V+.19 CON-LEVEL4-I+/V+.20 ; also sheet 1,2,3,4,5,7,9
I+1_1: CON-LEVEL1-I+/V+.4 ; also sheet 4
I+1_2: CON-LEVEL2-I+/V+.4 ; also sheet 4
I+1_3: CON-LEVEL3-I+/V+.4 ; also sheet 4
I+1_4: CON-LEVEL4-I+/V+.4 ; also sheet 4
I+3_1: CON-LEVEL1-I+/V+.6 ; also sheet 4
I+3_2: CON-LEVEL2-I+/V+.6 ; also sheet 4
I+3_3: CON-LEVEL3-I+/V+.6 ; also sheet 4
I+3_4: CON-LEVEL4-I+/V+.6 ; also sheet 4
I+5_1: CON-LEVEL1-I+/V+.8 ; also sheet 4
I+5_2: CON-LEVEL2-I+/V+.8 ; also sheet 4
I+5_3: CON-LEVEL3-I+/V+.8 ; also sheet 4
I+5_4: CON-LEVEL4-I+/V+.8 ; also sheet 4
I+7_1: CON-LEVEL1-I+/V+.10 ; also sheet 4
I+7_2: CON-LEVEL2-I+/V+.10 ; also sheet 4
I+7_3: CON-LEVEL3-I+/V+.10 ; also sheet 4
I+7_4: CON-LEVEL4-I+/V+.10 ; also sheet 4
I+9_1: CON-LEVEL1-I+/V+.12 ; also sheet 4
I+9_2: CON-LEVEL2-I+/V+.12 ; also sheet 4
I+9_3: CON-LEVEL3-I+/V+.12 ; also sheet 4
I+9_4: CON-LEVEL4-I+/V+.12 ; also sheet 4
I+11_1: CON-LEVEL1-I+/V+.14 ; also sheet 4
I+11_2: CON-LEVEL2-I+/V+.14 ; also sheet 4
I+11_3: CON-LEVEL3-I+/V+.14 ; also sheet 4
I+11_4: CON-LEVEL4-I+/V+.14 ; also sheet 4
I+13_1: CON-LEVEL1-I+/V+.16 ; also sheet 4
I+13_2: CON-LEVEL2-I+/V+.16 ; also sheet 4
I+13_3: CON-LEVEL3-I+/V+.16 ; also sheet 4
I+13_4: CON-LEVEL4-I+/V+.16 ; also sheet 4
I+15_1: CON-LEVEL1-I+/V+.18 ; also sheet 4
I+15_2: CON-LEVEL2-I+/V+.18 ; also sheet 4
I+15_3: CON-LEVEL3-I+/V+.18 ; also sheet 4
I+15_4: CON-LEVEL4-I+/V+.18 ; also sheet 4
V+1_1: CON-LEVEL1-I+/V+.3 ; also sheet 5
V+1_2: CON-LEVEL2-I+/V+.3 ; also sheet 5
V+1_3: CON-LEVEL3-I+/V+.3 ; also sheet 5
V+1_4: CON-LEVEL4-I+/V+.3 ; also sheet 5
V+3_1: CON-LEVEL1-I+/V+.5 ; also sheet 5
V+3_2: CON-LEVEL2-I+/V+.5 ; also sheet 5
V+3_3: CON-LEVEL3-I+/V+.5 ; also sheet 5
V+3_4: CON-LEVEL4-I+/V+.5 ; also sheet 5
V+5_1: CON-LEVEL1-I+/V+.7 ; also sheet 5
V+5_2: CON-LEVEL2-I+/V+.7 ; also sheet 5
V+5_3: CON-LEVEL3-I+/V+.7 ; also sheet 5
V+5_4: CON-LEVEL4-I+/V+.7 ; also sheet 5
V+7_1: CON-LEVEL1-I+/V+.9 ; also sheet 5
V+7_2: CON-LEVEL2-I+/V+.9 ; also sheet 5
V+7_3: CON-LEVEL3-I+/V+.9 ; also sheet 5
V+7_4: CON-LEVEL4-I+/V+.9 ; also sheet 5
V+9_1: CON-LEVEL1-I+/V+.11 ; also sheet 5
V+9_2: CON-LEVEL2-I+/V+.11 ; also sheet 5
V+9_3: CON-LEVEL3-I+/V+.11 ; also sheet 5
V+9_4: CON-LEVEL4-I+/V+.11 ; also sheet 5
V+11_1: CON-LEVEL1-I+/V+.13 ; also sheet 5
V+11_2: CON-LEVEL2-I+/V+.13 ; also sheet 5
V+11_3: CON-LEVEL3-I+/V+.13 ; also sheet 5
V+11_4: CON-LEVEL4-I+/V+.13 ; also sheet 5
V+13_1: CON-LEVEL1-I+/V+.15 ; also sheet 5
V+13_2: CON-LEVEL2-I+/V+.15 ; also sheet 5
V+13_3: CON-LEVEL3-I+/V+.15 ; also sheet 5
V+13_4: CON-LEVEL4-I+/V+.15 ; also sheet 5
V+15_1: CON-LEVEL1-I+/V+.17 ; also sheet 5
V+15_2: CON-LEVEL2-I+/V+.17 ; also sheet 5
V+15_3: CON-LEVEL3-I+/V+.17 ; also sheet 5
V+15_4: CON-LEVEL4-I+/V+.17 ; also sheet 5

## Sheet 7 of 9: Electrode Connections I- and V-
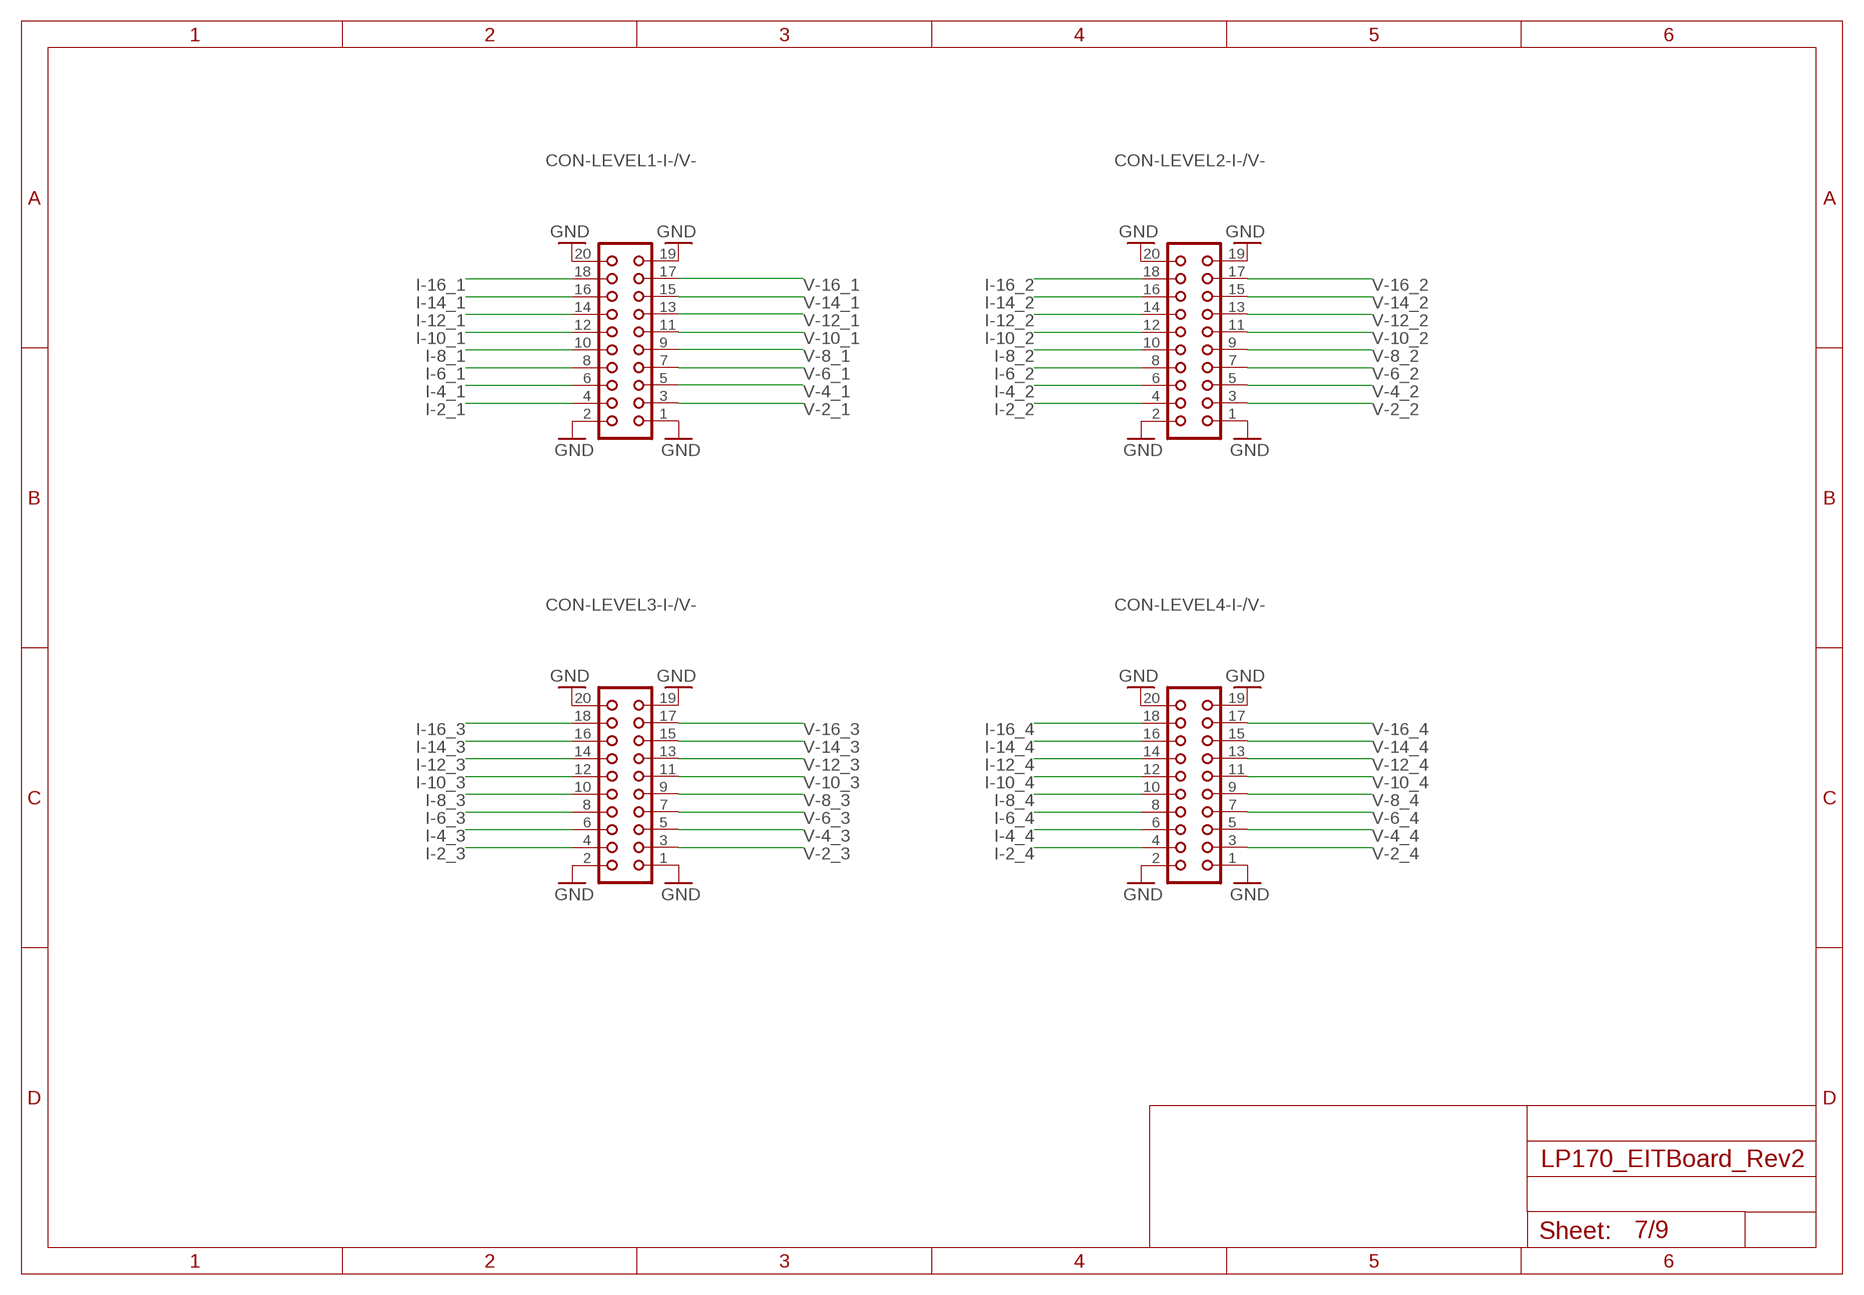
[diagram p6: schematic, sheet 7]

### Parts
CON-LEVEL1-I-/V-  CON20  [CON20]
CON-LEVEL2-I-/V-  CON20  [CON20]
CON-LEVEL3-I-/V-  CON20  [CON20]
CON-LEVEL4-I-/V-  CON20  [CON20]

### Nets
GND: CON-LEVEL1-I-/V-.1 CON-LEVEL1-I-/V-.2 CON-LEVEL1-I-/V-.19 CON-LEVEL1-I-/V-.20 CON-LEVEL2-I-/V-.1 CON-LEVEL2-I-/V-.2 CON-LEVEL2-I-/V-.19 CON-LEVEL2-I-/V-.20 CON-LEVEL3-I-/V-.1 CON-LEVEL3-I-/V-.2 CON-LEVEL3-I-/V-.19 CON-LEVEL3-I-/V-.20 CON-LEVEL4-I-/V-.1 CON-LEVEL4-I-/V-.2 CON-LEVEL4-I-/V-.19 CON-LEVEL4-I-/V-.20 ; also sheet 1,2,3,4,5,6,9
I-2_1: CON-LEVEL1-I-/V-.4 ; also sheet 4
I-2_2: CON-LEVEL2-I-/V-.4 ; also sheet 4
I-2_3: CON-LEVEL3-I-/V-.4 ; also sheet 4
I-2_4: CON-LEVEL4-I-/V-.4 ; also sheet 4
I-4_1: CON-LEVEL1-I-/V-.6 ; also sheet 4
I-4_2: CON-LEVEL2-I-/V-.6 ; also sheet 4
I-4_3: CON-LEVEL3-I-/V-.6 ; also sheet 4
I-4_4: CON-LEVEL4-I-/V-.6 ; also sheet 4
I-6_1: CON-LEVEL1-I-/V-.8 ; also sheet 4
I-6_2: CON-LEVEL2-I-/V-.8 ; also sheet 4
I-6_3: CON-LEVEL3-I-/V-.8 ; also sheet 4
I-6_4: CON-LEVEL4-I-/V-.8 ; also sheet 4
I-8_1: CON-LEVEL1-I-/V-.10 ; also sheet 4
I-8_2: CON-LEVEL2-I-/V-.10 ; also sheet 4
I-8_3: CON-LEVEL3-I-/V-.10 ; also sheet 4
I-8_4: CON-LEVEL4-I-/V-.10 ; also sheet 4
I-10_1: CON-LEVEL1-I-/V-.12 ; also sheet 4
I-10_2: CON-LEVEL2-I-/V-.12 ; also sheet 4
I-10_3: CON-LEVEL3-I-/V-.12 ; also sheet 4
I-10_4: CON-LEVEL4-I-/V-.12 ; also sheet 4
I-12_1: CON-LEVEL1-I-/V-.14 ; also sheet 4
I-12_2: CON-LEVEL2-I-/V-.14 ; also sheet 4
I-12_3: CON-LEVEL3-I-/V-.14 ; also sheet 4
I-12_4: CON-LEVEL4-I-/V-.14 ; also sheet 4
I-14_1: CON-LEVEL1-I-/V-.16 ; also sheet 4
I-14_2: CON-LEVEL2-I-/V-.16 ; also sheet 4
I-14_3: CON-LEVEL3-I-/V-.16 ; also sheet 4
I-14_4: CON-LEVEL4-I-/V-.16 ; also sheet 4
I-16_1: CON-LEVEL1-I-/V-.18 ; also sheet 4
I-16_2: CON-LEVEL2-I-/V-.18 ; also sheet 4
I-16_3: CON-LEVEL3-I-/V-.18 ; also sheet 4
I-16_4: CON-LEVEL4-I-/V-.18 ; also sheet 4
V-2_1: CON-LEVEL1-I-/V-.3 ; also sheet 5
V-2_2: CON-LEVEL2-I-/V-.3 ; also sheet 5
V-2_3: CON-LEVEL3-I-/V-.3 ; also sheet 5
V-2_4: CON-LEVEL4-I-/V-.3 ; also sheet 5
V-4_1: CON-LEVEL1-I-/V-.5 ; also sheet 5
V-4_2: CON-LEVEL2-I-/V-.5 ; also sheet 5
V-4_3: CON-LEVEL3-I-/V-.5 ; also sheet 5
V-4_4: CON-LEVEL4-I-/V-.5 ; also sheet 5
V-6_1: CON-LEVEL1-I-/V-.7 ; also sheet 5
V-6_2: CON-LEVEL2-I-/V-.7 ; also sheet 5
V-6_3: CON-LEVEL3-I-/V-.7 ; also sheet 5
V-6_4: CON-LEVEL4-I-/V-.7 ; also sheet 5
V-8_1: CON-LEVEL1-I-/V-.9 ; also sheet 5
V-8_2: CON-LEVEL2-I-/V-.9 ; also sheet 5
V-8_3: CON-LEVEL3-I-/V-.9 ; also sheet 5
V-8_4: CON-LEVEL4-I-/V-.9 ; also sheet 5
V-10_1: CON-LEVEL1-I-/V-.11 ; also sheet 5
V-10_2: CON-LEVEL2-I-/V-.11 ; also sheet 5
V-10_3: CON-LEVEL3-I-/V-.11 ; also sheet 5
V-10_4: CON-LEVEL4-I-/V-.11 ; also sheet 5
V-12_1: CON-LEVEL1-I-/V-.13 ; also sheet 5
V-12_2: CON-LEVEL2-I-/V-.13 ; also sheet 5
V-12_3: CON-LEVEL3-I-/V-.13 ; also sheet 5
V-12_4: CON-LEVEL4-I-/V-.13 ; also sheet 5
V-14_1: CON-LEVEL1-I-/V-.15 ; also sheet 5
V-14_2: CON-LEVEL2-I-/V-.15 ; also sheet 5
V-14_3: CON-LEVEL3-I-/V-.15 ; also sheet 5
V-14_4: CON-LEVEL4-I-/V-.15 ; also sheet 5
V-16_1: CON-LEVEL1-I-/V-.17 ; also sheet 5
V-16_2: CON-LEVEL2-I-/V-.17 ; also sheet 5
V-16_3: CON-LEVEL3-I-/V-.17 ; also sheet 5
V-16_4: CON-LEVEL4-I-/V-.17 ; also sheet 5

## Sheet 8 of 9: Rev.History
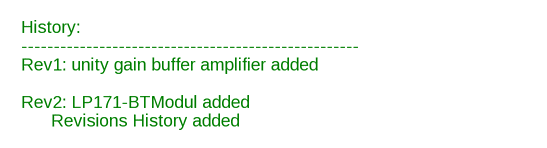
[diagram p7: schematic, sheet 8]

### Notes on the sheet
- History:
  ----------------------------------------------------
  Rev1: unity gain buffer amplifier added
  
  Rev2: LP171-BTModul added
        Revisions History added

## Sheet 9 of 9: BT Modul
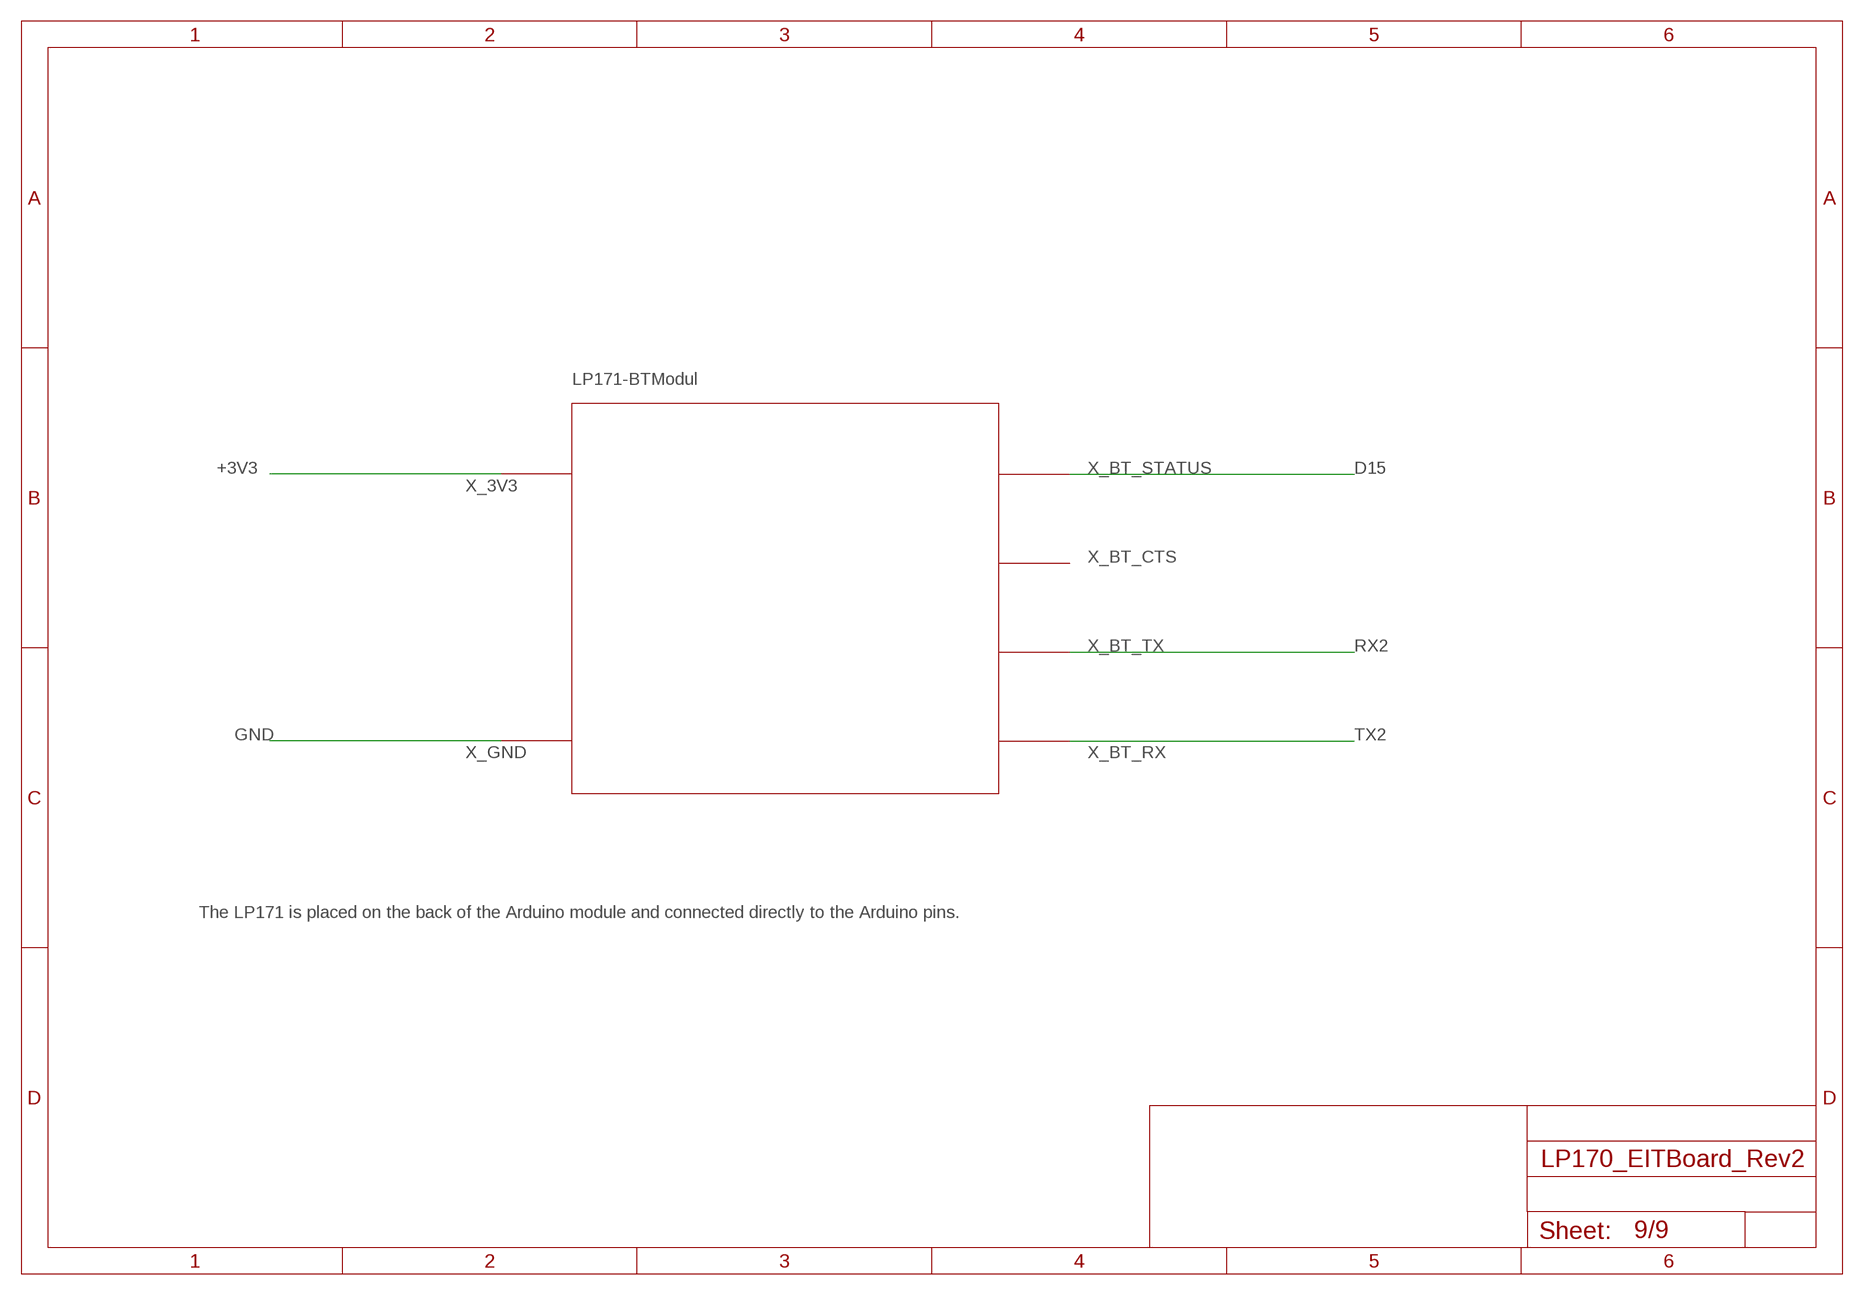
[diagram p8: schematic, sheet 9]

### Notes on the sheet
- LP171-BTModul
- X_BT_STATUS
- X_3V3
- X_BT_CTS
- X_BT_TX
- X_GND | X_BT_RX
- The LP171 is placed on the back of the Arduino module and connected directly to the Arduino pins.

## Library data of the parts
1V65 3V3 +5V -5V G GND GND70 HP I+ I- INST MCLK SCL SDA T1 V+ V- VIN VOUT = testpad:PTR1: TEST PIN
C201-C204 C301-C306 C401-C408 C501-C508 = rcl:C-EU: CAPACITOR, European symbol
CON-LEVEL1-I+/V+ CON-LEVEL1-I-/V- CON-LEVEL2-I+/V+ CON-LEVEL2-I-/V- CON-LEVEL3-I+/V+ CON-LEVEL3-I-/V- CON-LEVEL4-I+/V+ CON-LEVEL4-I-/V- = con-harting:CON20: CONNECTOR; OC_FARNELL: unknown; OC_NEWARK: unknown
D201 = SamacSys_Parts:STPS1L40U: STMicroelectronics 40V 1A, Diode, 2-Pin DO-214AA STPS1L40U; DESCRIPTION: STMicroelectronics 40V 1A, Diode, 2-Pin DO-214AA STPS1L40U; HEIGHT: 2.65mm; MANUFACTURER_NAME: STMicroelectronics; MANUFACTURER_PART_NUMBER: STPS1L40U; RS_PART_NUMBER: 4858077P; RS_PRICE-STOCK: http://uk.rs-online.com/web/p/products/4858077P
IC201 = SamacSys_Parts:DCWN03E-15: Module DC-DC 5VIN 2-OUT 15V/-15V 0.1A/-0.1A 3W 8-Pin DIP Module Source: Datasheet; ALLIED_NUMBER: 71028252; DESCRIPTION: Module DC-DC 5VIN 2-OUT 15V/-15V 0.1A/-0.1A 3W 8-Pin DIP Module; HEIGHT: 10.2mm; MANUFACTURER_NAME: Mean Well; MANUFACTURER_PART_NUMBER: DCWN03E-15
IC301 = SamacSys_Parts:AD5933WYRSZ-REEL7: Data Acquisition ADCs/DACs - Specialized 12bit 1 MSPS, Impedance Converter Source: Datasheet; DESCRIPTION: Data Acquisition ADCs/DACs - Specialized 12bit 1 MSPS, Impedance Converter; HEIGHT: 2mm; MANUFACTURER_NAME: Analog Devices; MANUFACTURER_PART_NUMBER: AD5933WYRSZ-REEL7
IC302 = linear:TL084: OP AMP
IC303 = linear:LMV321?*: General Purpose, Low Voltage, Rail-to-Rail Output Operational Amplifiers Source: http://www.national.com/mpf/LM/LMV321.html http://www.national.com/dt/lmv_qual.pdf
IC401-IC404 IC501-IC504 = SamacSys_Parts:DG1206ETJ+: Low-Leakage, Single 16-Channel and Dual 8-Channel, Analog Multiplexer, 32 TQFN Source: Datasheet; DESCRIPTION: Low-Leakage, Single 16-Channel and Dual 8-Channel, Analog Multiplexer, 32 TQFN; HEIGHT: 0.8mm; MANUFACTURER_NAME: Analog Devices; MANUFACTURER_PART_NUMBER: DG1206ETJ+
MEGA_CON1-MEGA_CON5 = adafruit:PINHD-1X8: PIN HEADER
MEGA_CON6 = adafruit:PINHD-1X10: Pin header 1x10 0.1" spacing With round pins
MEGA_CON7 = pinhead:PINHD-2X18: PIN HEADER
PWR = pinhead-2:PINHD-1X02: PIN HEADER
R301-R316 = rcl:R-EU_: RESISTOR, European symbol
T301 T302 = SamacSys_Parts:BSS138LT3G: MOSFET N-Channel 50V 0.2A SOT23 ON Semiconductor BSS138LT3G N-channel MOSFET Transistor, 0.2 A, 50 V, 3-Pin SOT-23 Source: Datasheet; ALLIED_NUMBER: 70339451; DESCRIPTION: MOSFET N-Channel 50V 0.2A SOT23 ON Semiconductor BSS138LT3G N-channel MOSFET Transistor, 0.2 A, 50 V, 3-Pin SOT-23; HEIGHT: 1.11mm; MANUFACTURER_NAME: onsemi; MANUFACTURER_PART_NUMBER: BSS138LT3G; RS_PART_NUMBER: 6900136P; RS_PRICE-STOCK: http://uk.rs-online.com/web/p/products/6900136P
